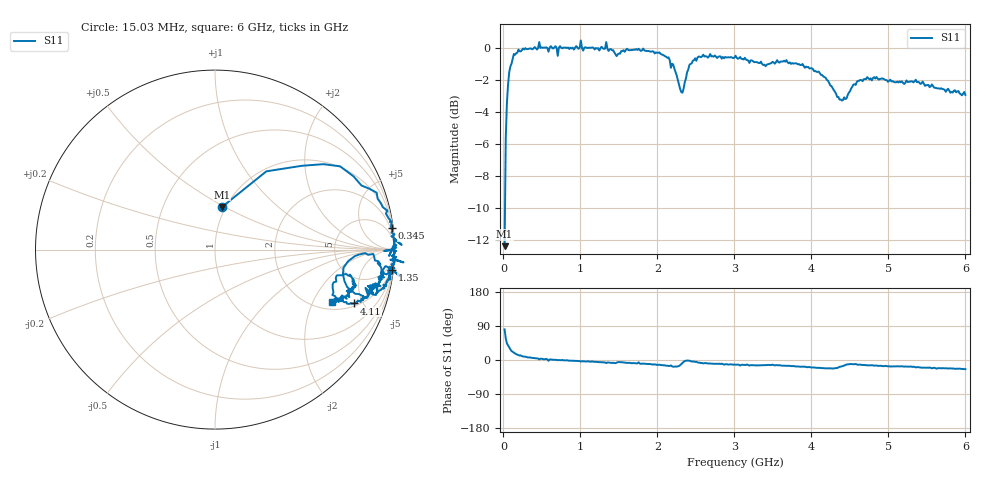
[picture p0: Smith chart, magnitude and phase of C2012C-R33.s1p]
!	Network	Analyzer	HP8753E.07.74:	Oct	30	2002	Serial	No.	JP38451487
!	Hewlett-Packard
!	7	Sep	2009	12:24:09
!	Frequency	S11
#	HZ	S	RI	R	50
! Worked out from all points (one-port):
!   400 points, 15.03 MHz to 6 GHz, reference 50 ohm
!   lowest |S11| = -12.4 dB at 15.03 MHz (marker M1), VSWR 1.63, Z = 48 + j24.2 ohm
!   |S11| at or under -10 dB: start of sweep to 20.36 MHz
!   S11 on the Smith chart (normalised r, x): 15.03 MHz: 0.96, +0.48; 345 MHz: 1, +16; 1.35 GHz: 1, -17; 4.11 GHz: 2.20, -4.28; 6 GHz: 2.39, -2.81
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1.502992e7  0.0384 0.237
3.002985e7  0.286 0.436
4.502978e7  0.484 0.467
1.050295e8  0.816 0.357
1.95029e8  0.961 0.217
3.450283e8  0.986 0.12
4.650277e8  1.04 0.0264
5.550272e8  1 0.0524
5.850271e8  0.97 -0.0351
6.00027e8  0.999 0.0245
7.050265e8  0.942 -0.00717
7.650262e8  0.995 0.00226
1.005025e9  1.05 -0.0714
1.035025e9  0.977 -0.0564
1.350023e9  0.986 -0.114
1.515022e9  0.953 -0.0927
2.02502e9  0.943 -0.211
2.265019e9  0.759 -0.228
2.325018e9  0.716 -0.101
2.385018e9  0.837 -0.0196
2.535017e9  0.93 -0.118
3.015015e9  0.921 -0.203
3.765011e9  0.857 -0.244
4.110009e9  0.776 -0.3
4.335008e9  0.654 -0.253
4.515007e9  0.732 -0.136
5.265004e9  0.746 -0.235
6e9  0.65 -0.29
